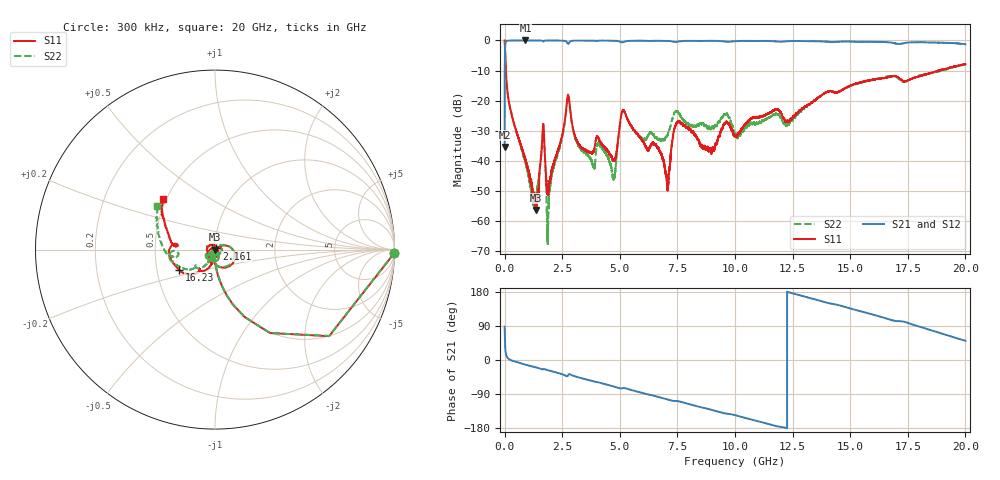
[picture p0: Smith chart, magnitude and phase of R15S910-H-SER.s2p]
!{R15S910}
!Johanson Technology Inc.
!www.johansontechnology.com
!Test Board Conditions:
!Substrate Type  RO4350B
!Substrate Thickness  20 mil
!Substrate Dk  3.66
!TL Type: GCPW
!TL Trace Width  34 mil
!TL Gap  10 mil
!Electrode orientation  Horizontal
!DUT TOPOLOGY	SERIES
!Mounting Pad LxW  26x52 mil
! Created Sat Feb  6 14:37:46 2021
# hz S ma R 50
! 2 Port Network Data from SP1.SP block
! freq  magS11  angS11  magS21  angS21  magS12  angS12  magS22  angS22
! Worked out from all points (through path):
!   20001 points, 300 kHz to 20 GHz, reference 50 ohm
!   highest |S21| = 0.00 dB at 906.3 MHz (marker M1); lowest = -35.4 dB at 300 kHz (marker M2)
!   group delay of S21, straight-line fit = 42.6 ps
!   lowest |S11| = -56.3 dB at 1.362 GHz (marker M3), VSWR 1.00, Z = 50.1 - j0.0561 ohm
!   |S11| at or under -10 dB: 52.8 MHz to 18.83 GHz (18.78 GHz wide, 199 % of centre); 18.83081 GHz to 18.8326 GHz (1.793 MHz wide, 0.00952 % of centre); 18.83662 GHz to 18.83892 GHz (2.306 MHz wide, 0.0122 % of centre)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
!   |S22| runs from -68.4 to 0.0 dB; largest |S21 - S12| = 0.015
!   S11 on the Smith chart (normalised r, x): 300 kHz: 7, -96; 2.161 GHz: 1.02, +0.01; 16.23 GHz: 0.65, -0.15; 20 GHz: 0.48, +0.32
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300000  0.9985 -1.2  0.01696 88.1  0.01702 88.8  0.9975 -1.1
1.143e8  0.1529 -82.7  0.9876 7.0  0.9875 7.0  0.1536 -82.8
9.063e8  0.01012 -95.9  0.9999 -12.2  0.9979 -12.3  0.009474 -111.1
1.3623e9  0.001529 -21.5  0.9982 -19.6  0.9984 -19.5  0.002544 123.4
1.6483e9  0.02931 28.6  0.9814 -25.0  0.9815 -25.0  0.02809 31.0
1.8873e9  0.002746 -8.5  0.9971 -27.1  0.9971 -27.2  0.0006756 102.5
2.1613e9  0.009825 39.3  0.9969 -31.6  0.9969 -31.6  0.0086 63.1
2.7543e9  0.1255 -35.4  0.8765 -40.6  0.8768 -40.5  0.1183 -36.0
3.3343e9  0.01615 -104.4  0.9955 -47.9  0.9951 -47.9  0.01499 -150.3
4.1233e9  0.02143 -113.8  0.9923 -59.8  0.9924 -59.8  0.01832 -154.2
4.7343e9  0.01045 -96.5  0.9896 -69.9  0.9896 -69.9  0.004997 -116.8
5.1643e9  0.06923 -114.8  0.9409 -73.8  0.9403 -73.8  0.07034 -113.2
6.6673e9  0.0164 135.7  0.989 -97.4  0.9888 -97.4  0.02221 -129.5
7.0613e9  0.00403 53.2  0.9825 -104.0  0.9824 -104.0  0.0262 -101.0
7.5203e9  0.04427 -171.6  0.9549 -108.5  0.9557 -108.5  0.06514 -142.3
8.9123e9  0.01617 46.7  0.9858 -130.5  0.9864 -130.5  0.03382 -117.1
9.5903e9  0.04316 -91.2  0.9575 -141.3  0.9577 -141.2  0.05896 -102.0
1.00003e10  0.02674 -114.1  0.9724 -145.5  0.9727 -145.5  0.02863 -110.4
1.33343e10  0.09245 -105.3  0.9731 162.3  0.9742 162.3  0.09416 -119.3
1.62253e10  0.23 -150.8  0.9466 115.7  0.9444 115.7  0.2316 -158.5
1.66673e10  0.244 -163.7  0.9326 107.7  0.9201 107.6  0.2549 -166.1
2e10  0.4034 135.7  0.8643 50.8  0.8567 50.5  0.4029 142.8
